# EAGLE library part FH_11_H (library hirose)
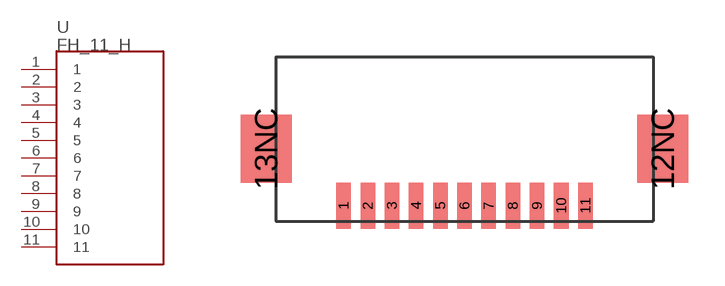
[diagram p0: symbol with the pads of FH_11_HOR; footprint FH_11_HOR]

Designator prefix -

## FH_11_H  [FH_11_HOR]
1  1
2  2
3  3
4  4
5  5
6  6
7  7
8  8
9  9
10  10
11  11

## Footprint FH_11_HOR (pad centres in mm)
smd 0.6 x 1.9: 1 -5,0.65; 2 -4,0.65; 3 -3,0.65; 4 -2,0.65; 5 -1,0.65; 6 0,0.65; 7 1,0.65; 8 2,0.65; 9 3,0.65; 10 4,0.65; 11 5,0.65
smd 2.1 x 2.8: 12NC 8.2,3; 13NC -8.2,3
